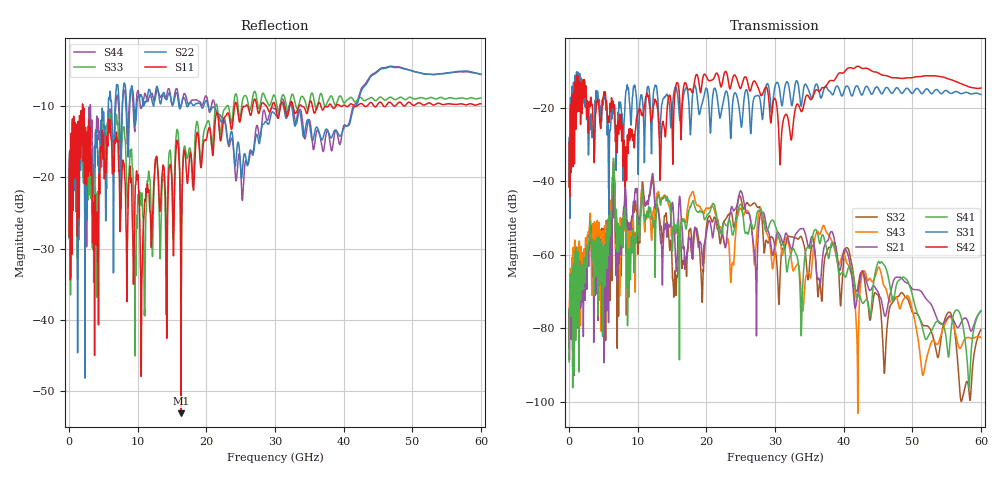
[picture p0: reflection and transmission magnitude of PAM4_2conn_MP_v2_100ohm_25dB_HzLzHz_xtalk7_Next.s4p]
! Info: Touchstone file created by Circ.  Input file=FAB50GbE_2conn_Midplane_Examax_Topo2_v2_100ohm_25dB_HzLzHz.circ
# Hz S RI R 50
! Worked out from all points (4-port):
!   6000 points, 10 MHz to 60 GHz, reference 50 ohm
!   strongest paths, dB at 10 MHz, 15.01 GHz, 30.01 GHz, 45.01 GHz, 60 GHz:
!     S42: -41.6, -24.7, -17.5, -10.5, -14.7
!     S31: -41.5, -21.1, -14.1, -14.6, -16.4
!     S41: -89.2, -56.8, -51.9, -62.1, -75.3
!     S21: -75.8, -46.0, -56.8, -70.1, -75.4
!     S43: -77.6, -52.8, -58.7, -63.6, -82.6
!     S32: -81.0, -63.1, -58.2, -71.0, -80.4
!   lowest |S11| = -53.1 dB at 16.32 GHz (marker M1), VSWR 1.00, Z = 50.1 + j0.212 ohm
!   |S11| at or under -10 dB: start of sweep to 1.951 GHz; 1.996 GHz to 24.12 GHz (22.13 GHz wide, 169 % of centre); 24.48 GHz to 25.69 GHz (1.216 GHz wide, 4.85 % of centre)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
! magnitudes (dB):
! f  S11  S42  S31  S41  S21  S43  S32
! 10 MHz  -28.3  -41.6  -41.5  -89.2  -75.8  -77.6  -81.0
! 1.32 GHz  -12.1  -11.4  -10.3  -61.2  -63.1  -60.5  -62.2
! 6.42 GHz  -17.2  -18.7  -21.0  -35.4  -42.9  -35.7  -43.6
! 8.68 GHz  -20.9  -26.9  -15.1  -60.9  -51.3  -55.9  -52.3
! 16.32 GHz  -53.1  -28.5  -21.8  -51.4  -49.3  -51.0  -57.8
! 24.89 GHz  -12.2  -14.7  -21.9  -46.4  -42.9  -47.5  -44.0
! 60 GHz  -9.7  -14.7  -16.4  -75.3  -75.4  -82.6  -80.4
